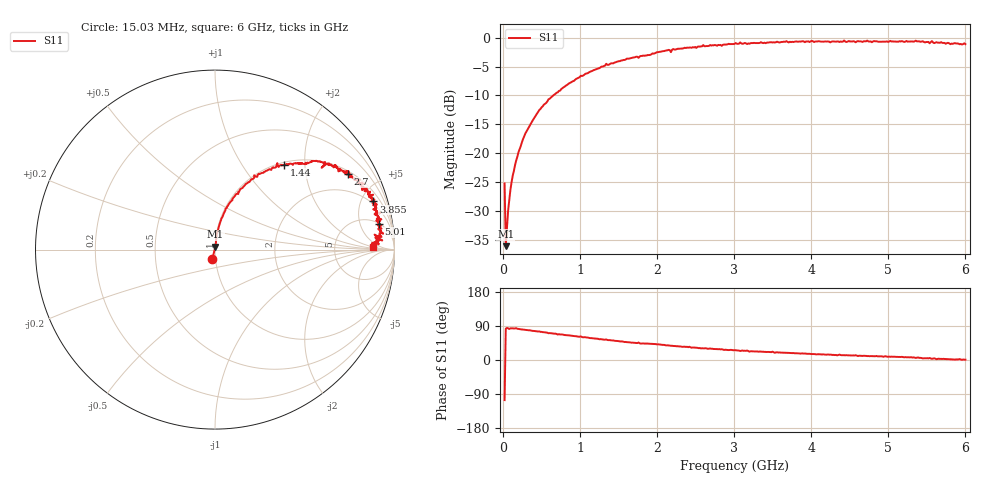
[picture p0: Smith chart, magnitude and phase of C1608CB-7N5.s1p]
!	Network	Analyzer	HP8753E.07.74:	Oct	30	2002	Serial	No.	JP38451487
!	Hewlett-Packard
!	27	Aug	2009	16:26:31
!	Frequency	S11
#	HZ	S	RI	R	50
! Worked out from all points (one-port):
!   400 points, 15.03 MHz to 6 GHz, reference 50 ohm
!   lowest |S11| = -36.1 dB at 30.03 MHz (marker M1), VSWR 1.03, Z = 50.2 + j1.57 ohm
!   |S11| at or under -10 dB: start of sweep to 647 MHz
!   S11 on the Smith chart (normalised r, x): 15.03 MHz: 0.97, -0.10; 1.44 GHz: 1.05, +1.56; 2.7 GHz: 1.11, +3.44; 3.855 GHz: 1.74, +6.27; 5.01 GHz: 5, +10; 6 GHz: 15, +2
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1.502992e7  -0.015 -0.0527
3.002985e7  0.00203 0.0156
6.00297e7  0.00349 0.0315
1.050295e8  0.00638 0.0556
1.650292e8  0.00891 0.0859
2.550287e8  0.0224 0.131
4.650277e8  0.059 0.229
7.650262e8  0.141 0.337
1.335023e9  0.347 0.482
1.440023e9  0.383 0.471
1.515022e9  0.41 0.473
2.265019e9  0.645 0.475
2.700016e9  0.741 0.422
3.015015e9  0.807 0.391
3.075015e9  0.832 0.365
3.165014e9  0.796 0.373
3.195014e9  0.82 0.331
3.495013e9  0.842 0.34
3.525012e9  0.858 0.296
3.765011e9  0.869 0.289
3.855011e9  0.883 0.268
4.515007e9  0.905 0.196
5.010005e9  0.914 0.144
5.265004e9  0.919 0.114
5.535002e9  0.889 0.0836
5.565002e9  0.932 0.0508
5.625002e9  0.912 0.0295
6e9  0.878 0.0129
